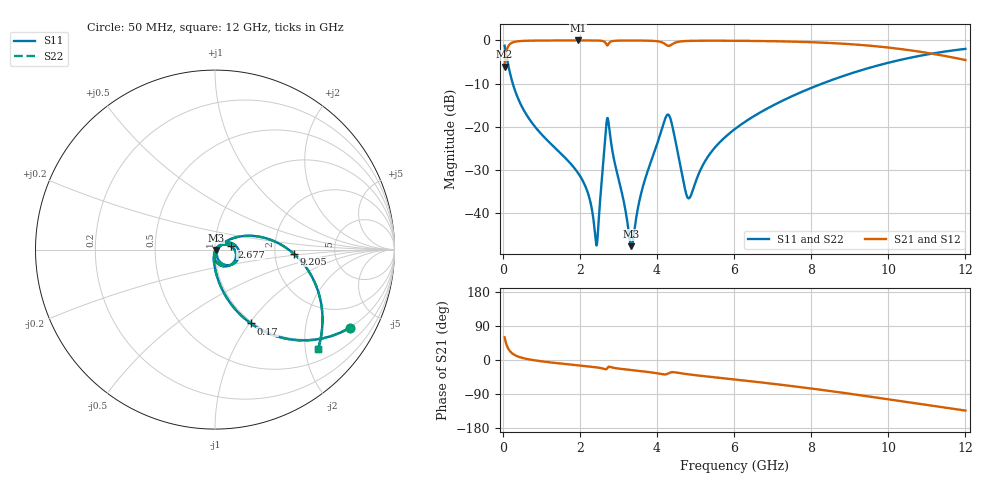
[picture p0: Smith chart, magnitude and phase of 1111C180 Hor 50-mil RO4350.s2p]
# GHz S MA R 50
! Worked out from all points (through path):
!   11951 points, 50 MHz to 12 GHz, reference 50 ohm
!   highest |S21| = -0.02 dB at 1.953 GHz (marker M1); lowest = -6.1 dB at 50 MHz (marker M2)
!   group delay of S21, straight-line fit = 32.4 ps
!   lowest |S11| = -47.6 dB at 3.339 GHz (marker M3), VSWR 1.01, Z = 50.4 - j0.196 ohm
!   |S11| at or under -10 dB: 262 MHz to 8.283 GHz (8.021 GHz wide, 188 % of centre)
!   |S22| runs from -47.6 to -1.2 dB; largest |S21 - S12| = 0
!   S11 on the Smith chart (normalised r, x): 50 MHz: 0.98, -3.46; 170 MHz: 0.98, -1.02; 2.677 GHz: 1.20, +0.04; 9.205 GHz: 2.55, -0.14; 12 GHz: 0.74, -2.27
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0.05  0.8684 -30.1  0.4956 59.9  0.4956 59.9  0.8684 -30.1
0.17  0.4575 -64.1  0.8887 25.8  0.8887 25.8  0.4575 -64.1
0.323  0.2606 -77.4  0.9648 12.5  0.9648 12.5  0.2606 -77.4
0.667  0.1276 -87.7  0.9909 1.9  0.9909 1.9  0.1276 -87.7
1.953  0.02936 -100.9  0.9978 -14.1  0.9978 -14.1  0.02936 -100.9
2.042  0.02542 -101.1  0.9978 -15.0  0.9978 -15.0  0.02542 -101.1
2.248  0.01512 -98.4  0.9974 -17.2  0.9974 -17.2  0.01512 -98.4
2.435  0.004246 -29.6  0.9957 -19.5  0.9957 -19.5  0.004246 -29.6
2.482  0.007295 21.2  0.9944 -20.2  0.9944 -20.2  0.007295 21.2
2.677  0.09329 10.8  0.9223 -24.5  0.9223 -24.5  0.09329 10.8
2.752  0.1063 -61.6  0.9203 -17.8  0.9203 -17.8  0.1063 -61.6
3.339  0.00418 -27.8  0.9956 -26.6  0.9956 -26.6  0.00418 -27.8
3.619  0.01909 43.5  0.9941 -29.8  0.9941 -29.8  0.01909 43.5
4.034  0.06948 34.2  0.9736 -35.6  0.9736 -35.6  0.06948 34.2
4.324  0.1336 -33.4  0.8662 -34.1  0.8662 -34.1  0.1336 -33.4
4.83  0.01492 -17.3  0.9858 -38.0  0.9858 -38.0  0.01492 -17.3
5.326  0.04549 37.0  0.9914 -43.8  0.9914 -43.8  0.04549 37.0
6.025  0.09464 35.1  0.9895 -51.5  0.9895 -51.5  0.09464 35.1
8.017  0.2839 13.3  0.9524 -75.5  0.9524 -75.5  0.2839 13.3
9.205  0.4386 -2.9  0.8912 -92.0  0.8912 -92.0  0.4386 -2.9
10.009  0.5523 -14.7  0.8254 -103.9  0.8254 -103.9  0.5523 -14.7
12  0.7982 -44.1  0.5926 -133.4  0.5926 -133.4  0.7982 -44.1
